PROGRAM MAIN

VAR	
(* 选择功能块，温度控制库有两个功能块版本 V1和 V2 ，系统通过默认选择 V1，V1为旧版本，已被淘汰 *)
	nSelectController	: UINT := 1;	
	
(* 激活系统触发条件 *)	
	bStart				: BOOL;			
END_VAR

(* 调用功能块V2，需将nSelectController从1切换为2 *)
IF bStart THEN
	       	nSelectController:= 2  ;   
			Controller_v2();		
END_IF;

END_PROGRAM
